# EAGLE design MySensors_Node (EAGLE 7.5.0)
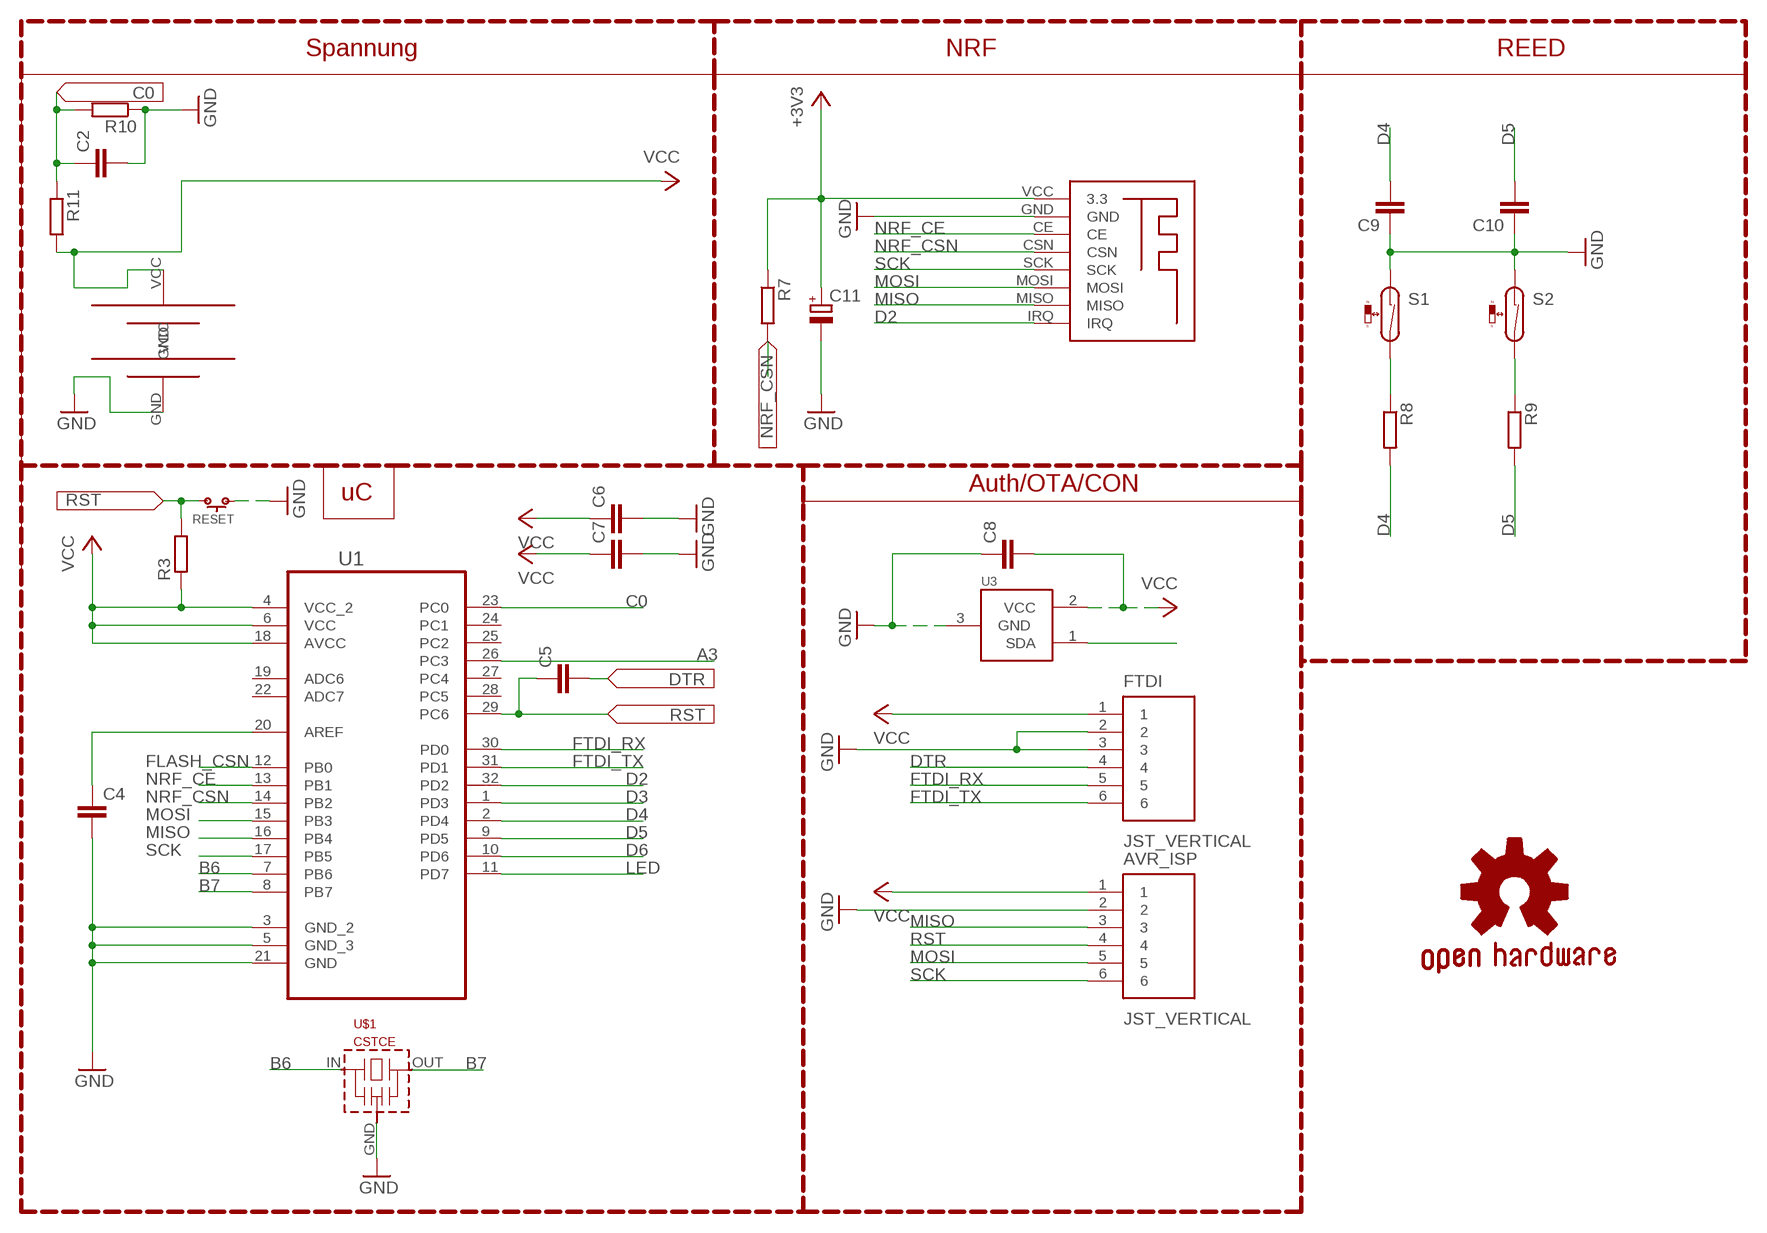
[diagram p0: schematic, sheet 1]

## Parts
AVR_ISP  JST_VERTICAL  [JST-6-SMD-VERT-1.0MM]
C2  C-EUC0805  [C0805]
C4  C-EUC0805  [C0805]
C5  C-EUC0805  [C0805]
C6  C-EUC0805  [C0805]
C7  C-EUC0805  [C0805]
C8  C-EUC0805  [C0805]
C9  C-EUC0805  [C0805]
C10  C-EUC0805  [C0805]
C11  CPOL-EUSANYO_SMD_C6  [SANYO-OSCON_SMD_C6]
FTDI  JST_VERTICAL  [JST-6-SMD-VERT-1.0MM]
GOLD_ORB_SM1  OSHWLOGO_GOLD_ORB_SM  [OSHW2]
R3  R-EU_R0805  [R0805]
R7  R-EU_R0805  [R0805]
R8  R-EU_R0805  [R0805]
R9  R-EU_R0805  [R0805]
R10  R-EU_R0805  [R0805]
R11  R-EU_R0805  [R0805]
RESET  SPST.B3U-1000P(M)  [B3U-1000P(M)]
S1  REED-SWITCH-MK6-5-C  [MK6-5]
S2  REED-SWITCH-MK6-5-C  [MK6-5]
U1  ATMEGA328P-AU  [QFP80P900X900X120-32N]
U3  IC_ATSHA204A_CRYPT  [SOT23-3]
U$1  CSTCE  [CSTCE]
U$2  NRF24SMD  [NRF24SMD]
U$3  AAA_HOLDER  [AAA_HOLDER]

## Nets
A3: U1.26(PC3) U3.1(SDA)
B6: U1.7(PB6) U$1.IN
B7: U1.8(PB7) U$1.OUT
C0: C2.1 R10.2 R11.1 U1.23(PC0)
D2: U1.32(PD2) U$2.IRQ
D3: U1.1(PD3)
D4: C9.2 R8.2 U1.2(PD4)
D5: C10.2 R9.2 U1.9(PD5)
D6: U1.10(PD6)
DTR: C5.2 FTDI.4
FLASH_CSN: U1.12(PB0)
FTDI_RX: FTDI.5 U1.30(PD0)
FTDI_TX: FTDI.6 U1.31(PD1)
GND: AVR_ISP.2 C2.2 C4.2 C6.2 C7.2 C8.1 C9.1 C10.1 C11.- FTDI.2 FTDI.3 R10.1 RESET.1 S1.1 S2.1 U1.3(GND_2) U1.5(GND_3) U1.21(GND) U3.3(GND) U$1.GND U$2.GND U$3.GND
LED: U1.11(PD7)
MISO: AVR_ISP.3 U1.16(PB4) U$2.MISO
MOSI: AVR_ISP.5 U1.15(PB3) U$2.MOSI
N$4: R8.1 S1.2
N$5: R9.1 S2.2
N$7: C4.1 U1.20(AREF)
NRF_CE: U1.13(PB1) U$2.CE
NRF_CSN: R7.2 U1.14(PB2) U$2.CSN
RST: AVR_ISP.4 C5.1 R3.2 RESET.2 U1.29(PC6)
SCK: AVR_ISP.6 U1.17(PB5) U$2.SCK
VCC: AVR_ISP.1 C6.1 C7.1 C8.2 C11.+ FTDI.1 R3.1 R7.1 R11.2 U1.4(VCC_2) U1.6(VCC) U1.18(AVCC) U3.2(VCC) U$2.VCC(3.3) U$3.VCC ; supply symbol labelled +3V3
Unconnected: U1.19(ADC6) U1.22(ADC7) U1.24(PC1) U1.25(PC2) U1.27(PC4) U1.28(PC5)

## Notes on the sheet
- Spannung | NRF | REED
- Auth/OTA/CON
- uC

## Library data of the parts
AVR_ISP FTDI = SparkFun-Connectors:JST_VERTICAL; PROD_ID: CONN-08249
C2 C4-C10 = rcl:C-EU: CAPACITOR, European symbol
C11 = rcl:CPOL-EU: POLARIZED CAPACITOR, European symbol
GOLD_ORB_SM1 = bfl:OSHWLOGO: These are Open-Source Hardware logos.
R3 R7-R11 = rcl:R-EU_: RESISTOR, European symbol
RESET = omron:SPST
S1 S2 = switch-reed:REED-SWITCH-: Reed Sensor; MF: MEDER; MPN: MK6-5-C; OC_FARNELL: 1079480
U1 = Atmel_By_element14_Batch_1-00:ATMEGA328P-AU: 8-bit Microcontroller with In-System Programmable Flash; MPN: ATMEGA328P-AU; OC_FARNELL: 1715486; OC_NEWARK: 14R4631; PACKAGE: TQFP-32; SUPPLIER: Atmel
U3 = TD-MySensors:IC_ATSHA204A_CRYPT
U$1 = murata-cstcc-cstce-cstcr-cstcv-resonators:CSTCE: Murata CSTCE Resonator - 3,2 x 1,3 mm
U$2 = NRF24_SMD:NRF24SMD
U$3 = Andi_lib:AAA_HOLDER

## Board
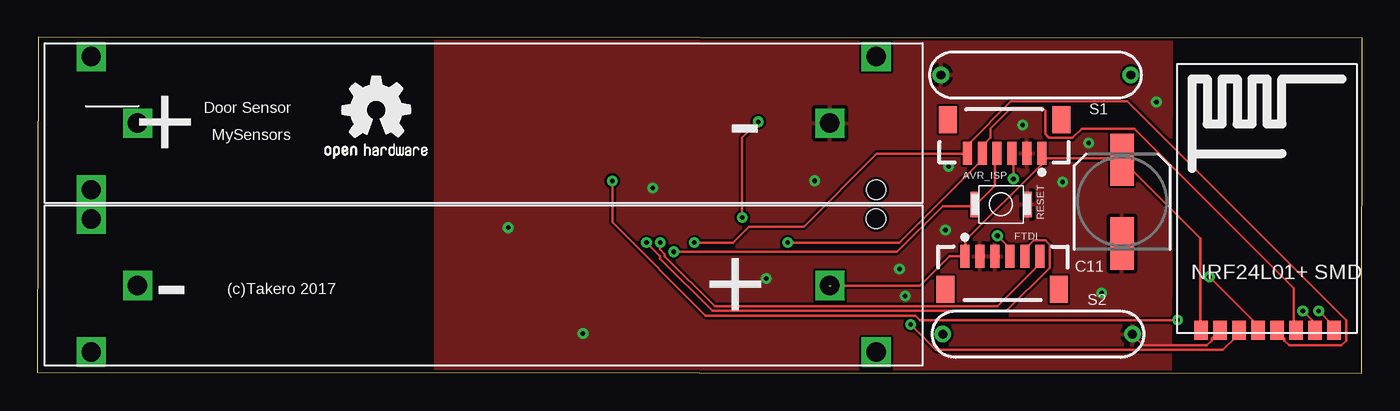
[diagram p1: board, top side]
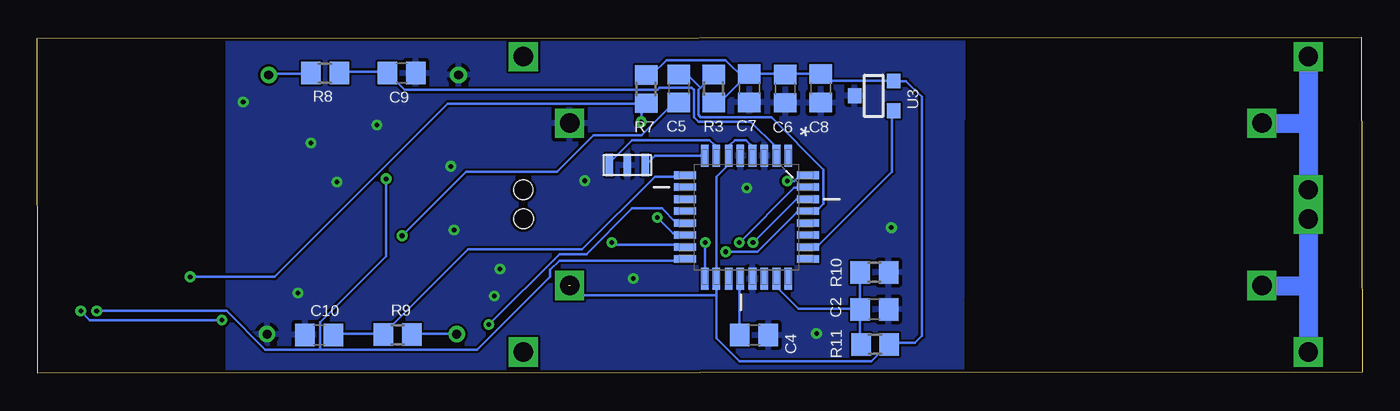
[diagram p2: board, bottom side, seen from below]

Size 88.6 x 22.47 mm. Coordinates in mm from the lower left corner, seen from the top.
Outline: 0.04,22.47 0,0.06 88.59,0 88.6,22.42 0.04,22.47
Copper layers (1*16): Top 0.035mm / dielectric 1.5mm / Bottom 0.035mm
Design rules "default *": minimum track width 6mil, minimum drill 12mil, track to track 6mil, track to pad 6mil, pad to pad 6mil, via to via 6mil, smd to smd 6mil, copper to edge 8mil, drill to drill 4mil, minimum pad ring 10mil, minimum via ring 8mil, stop-mask expansion 4mil, vias tented up to drill 12mil, thermal gap 10mil

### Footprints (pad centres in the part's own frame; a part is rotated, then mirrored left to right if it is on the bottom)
JST-6-SMD-VERT-1.0MM = smd 0.6 x 1.55: 1 -2.54,1.27; 2 -1.54,1.27; 3 -0.54,1.27; 4 0.46,1.27; 5 1.46,1.27; 6 2.46,1.27 | smd 1.2 x 1.8: P$1 -3.84,-0.955; P$2 3.76,-0.955
C0805 = smd 1.3 x 1.5: 1 -0.95,0; 2 0.95,0
SANYO-OSCON_SMD_C6 = smd 3.5 x 1.6: + 2.8,0; - -2.8,0
R0805 = smd 1.3 x 1.5: 1 -0.95,0; 2 0.95,0
B3U-1000P(M) = smd 0.6 x 1.7: 1 -1.75,0; 2 1.75,0
MK6-5 = drill 0.6 pad 1.016: 1 -6.35,0; 2 6.35,0
QFP80P900X900X120-32N = smd 1.473 x 0.508: 1 -4.115,2.794; 2 -4.115,2.007; 3 -4.115,1.194; 4 -4.115,0.406; 5 -4.115,-0.406; 6 -4.115,-1.194; 7 -4.115,-2.007; 8 -4.115,-2.794; 17 4.115,-2.794; 18 4.115,-2.007; 19 4.115,-1.194; 20 4.115,-0.406; 21 4.115,0.406; 22 4.115,1.194; 23 4.115,2.007; 24 4.115,2.794 | smd 0.508 x 1.473: 9 -2.794,-4.115; 10 -2.007,-4.115; 11 -1.194,-4.115; 12 -0.406,-4.115; 13 0.406,-4.115; 14 1.194,-4.115; 15 2.007,-4.115; 16 2.794,-4.115; 25 2.794,4.115; 26 2.007,4.115; 27 1.194,4.115; 28 0.406,4.115; 29 -0.406,4.115; 30 -1.194,4.115; 31 -2.007,4.115; 32 -2.794,4.115
SOT23-3 = smd 1 x 0.9: 1 -1,-1.3; 2 1,-1.3; 3 0,1.3
CSTCE = smd 0.5 x 1.5: GND 0,0; IN 1.2,0; OUT -1.2,0
NRF24SMD = smd 0.9 x 1.27: CE -1.27,-6.35; CSN 0,-6.35; GND -2.54,-6.35; IRQ 5.08,-6.35; MISO 3.81,-6.35; MOSI 2.54,-6.35; SCK 1.27,-6.35; VCC -3.81,-6.35
AAA_HOLDER = drill 1.3 pad 1.676 square: GND -5.35,27.75; P$1 5.5,-18.55; P$2 9.95,-21.65; P$3 1.05,-21.65; P$5 9.95,30.85; P$7 -5.35,-18.55; P$8 -0.9,-21.65; P$9 -9.8,-21.65; P$12 -9.8,30.85; VCC 5.5,27.75 | hole 1.3: -0.891,30.849; 1.051,30.842

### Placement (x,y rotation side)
AVR_ISP  64.65,16 180 top
C2  32.62,4.29 0 bottom
C4  40.66,2.56 0 bottom
C5  45.69,19.05 270 bottom
C6  38.58,19.05 270 bottom
C7  40.98,19.07 270 bottom
C8  36.2,19.05 90 bottom
C9  64.24,20.08 180 bottom
C10  69.75,2.57 0 bottom
C11  72.55,11.49 90 top
FTDI  64.57,6.57 0 top
GOLD_ORB_SM1  18.84,13.32 0 top
R3  43.37,19.05 90 bottom
R7  47.88,19.01 270 bottom
R8  69.37,20.08 0 bottom
R9  64.51,2.59 180 bottom
R10  32.62,6.75 180 bottom
R11  32.57,1.94 0 bottom
RESET  64.45,11.3 180 top
S1  66.78,19.95 0 top
S2  66.9,2.63 180 top
U1  41.18,10.45 270 bottom
U3  32.64,18.55 90 bottom
U$1  49.14,13.92 180 bottom
U$2  81.63,9.25 0 top
U$3  25.25,11.38 270 top

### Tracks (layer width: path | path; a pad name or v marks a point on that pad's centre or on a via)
A3
  Bottom 0.152: U3.1 31.44,17.43 31.44,13.47 36.32,8.59 36.93,8.59 U1.26
B6
  Bottom 0.152: U1.7 43.33,14.69 43.33,15.3 43.63,15.6 48.82,15.6 50.19,14.23 50.19,13.93 U$1.IN
B7
  Bottom 0.152: U1.8 44.09,14.54 47.29,14.54 47.9,13.93 U$1.OUT
C0
  Bottom 0.152: 33.58,4.33 37.69,4.33 39.06,5.7 39.06,6.31 U1.23 | R11.1 33.58,2.04 33.58,4.17 C2.1 33.58,4.33 | 33.58,4.33 33.58,6.61 R10.2
D2  (via drill 0.3)
  Top 0.152: v85.7,4.17 86.61,3.26 86.61,2.95 U$2.IRQ | v76.25,3.56 59.03,3.56 58.72,3.87 44.7,3.87 38.45,10.12 v38.45,12.86
  Bottom 0.152: v85.7,4.17 85.09,3.56 v76.25,3.56 | v38.45,12.86 37.99,12.86 37.69,13.16 37.08,13.16 U1.32
D4
  Bottom 0.152: U1.2 39.21,14.69 39.21,15.15 40.89,16.82 44.4,16.82 44.7,17.13 44.7,18.96 44.85,19.11 46.99,19.11 47.14,18.96 64.06,18.96 65.12,20.02 C9.2 65.27,20.18 68.32,20.18 R8.2
D5
  Bottom 0.152: U1.9 45.31,13.16 47.29,13.16 52.17,8.29 59.79,8.29 65.43,2.65 R9.2 65.58,2.65 68.78,2.65 C10.2
DTR  (via drill 0.3)
  Top 0.152: v64.21,9.2 64.97,8.44 64.97,7.98 FTDI.4
  Bottom 0.152: v64.21,9.2 59.94,13.47 53.84,13.47 51.41,15.91 48.21,15.91 46.07,18.04 45.77,18.04 C5.2
FTDI_RX  (via drill 0.3)
  Top 0.152: v40.74,8.75 41.65,7.83 41.65,7.68 45.16,4.17 64.82,4.17 67.71,7.07 67.71,8.59 67.41,8.9 66.65,8.9 66.04,8.29 66.04,7.98 FTDI.5
  Bottom 0.152: v40.74,8.75 37.84,11.64 37.08,11.64 U1.30
FTDI_TX  (via drill 0.3)
  Top 0.152: v41.65,8.75 41.65,8.29 41.96,7.98 41.96,7.83 45.31,4.48 64.21,4.48 66.95,7.22 66.95,7.83 FTDI.6
  Bottom 0.152: v41.65,8.75 37.99,12.4 37.08,12.4 U1.31
GND  (via drill 0.3)
  Top 0.152: U$2.GND 78.99,2.8 78.53,2.34 78.53,2.19 78.23,1.89 73.96,1.89 73.35,2.5 S2.1 | 63.14,7.83 FTDI.2
  Bottom 0.152: C7.2 41.04,18.19 41.1,18
  other vias: 36.49,2.68 31.48,9.74 41.15,12.4 51.98,12.88 68.57,12.8 74.83,18.15 70.3,15.39 65.89,16.61 71.19,5.39 60.94,13.85 60.73,9.6 57.66,6.97 48.75,6.35 58.04,5.18
  pour Bottom: 26.76,22.9 26.84,-0.95 75.79,-1.11 75.81,23.1
  pour Top: 26.64,22.92 26.64,-0.71 75.76,-0.96 75.83,23.16
MISO  (via drill 0.3)
  Top 0.152: v84.63,4.17 85.39,3.41 85.39,2.95 U$2.MISO | v65.27,13.01 65.27,14.69 AVR_ISP.3
  Bottom 0.152: v84.63,4.17 75.94,4.17 73.35,1.58 69.69,1.58 | 69.69,1.58 59.18,1.58 54.3,6.46 54.3,6.92 53.69,7.53 45.31,7.53 U1.16 | v65.27,13.01 65.27,7.83 69.69,3.41 69.69,1.58
MOSI  (via drill 0.3)
  Top 0.152: U$2.MOSI 84.02,2.95 84.02,5.7 73.35,16.37 69.85,16.37 69.24,15.76 69.23,15.76 67.66,15.76 67.4,16.02 67.4,17.55 67.2,17.75 65.14,17.75 63.75,16.36 63.75,15.76 63.29,15.3 63.29,14.84 AVR_ISP.5 63.14,14.69 63.14,14.23 57.65,8.75 v50.19,8.75
  Bottom 0.152: v50.19,8.75 50.03,8.59 45.31,8.59 U1.15
N$2
  Bottom 1.27: 3.59,21.18 3.6,21.18 3.6,1.43
N$3
  Bottom 1.27: 6.7,16.71 3.62,16.71 3.62,16.69
N$4
  Bottom 0.152: R8.1 70.46,20.02 73.05,20.02 S1.2
N$5
  Bottom 0.152: R9.1 63.45,2.65 60.55,2.65 S2.2
N$6
  Bottom 1.27: 6.7,5.87 3.66,5.87
N$7
  Bottom 0.152: U1.20 41.65,6.31 41.65,2.65 C4.1
NRF_CE  (via drill 0.3)
  Top 0.152: v58.42,3.26 60.09,1.58 79.3,1.58 80.21,2.5 80.21,2.8 U$2.CE
  Bottom 0.152: v58.42,3.26 53.69,7.98 51.86,7.98 48.82,11.03 46.83,11.03 45.92,10.12 45.31,10.12 U1.13
NRF_CSN  (via drill 0.3)
  Top 0.152: v78.38,6.46 81.58,3.26 81.58,2.95 U$2.CSN | v47.14,10.42 47.14,15.76 v48.21,16.82
  Bottom 0.152: v78.38,6.46 72.74,6.46 61.16,18.04 48.21,18.04 | 48.21,18.04 47.9,18.04 R7.2 48.21,18.04 | v47.14,10.42 46.07,9.35 45.31,9.35 U1.14 | 48.21,18.04 v48.21,16.82
RST  (via drill 0.3)
  Top 0.152: AVR_ISP.4 64.06,14.69 64.06,12.56 62.84,11.34 RESET.2 62.68,11.18 60.55,11.18 57.5,8.14 v42.57,8.14
  Bottom 0.152: 44.24,19.11 43.48,19.87 R3.2 | 44.24,19.11 44.4,18.96 44.4,17.28 44.24,17.13 39.52,17.13 36.01,13.62 36.01,11.34 36.47,10.88 36.93,10.88 U1.29 37.08,10.73 37.84,10.73 40.43,8.14 v42.57,8.14 | 44.24,19.11 45.01,19.87 45.61,19.87 C5.1
SCK  (via drill 0.3)
  Top 0.152: U$2.SCK 82.95,2.8 83.41,2.34 83.41,2.19 83.71,1.89 87.22,1.89 87.52,2.19 87.52,3.56 72.89,18.19 65.12,18.19 62.23,15.3 62.23,14.84 AVR_ISP.6 62.07,14.69 56.13,14.69 51.25,9.81 47.6,9.81 46.53,8.75 v43.94,8.75
  Bottom 0.152: v43.94,8.75 43.94,6.46 U1.17
VCC  (2 unrouted)
  Top 0.152: U$2.VCC 77.77,2.95 77.77,9.05 72.59,14.23 C11.+ 72.44,14.38 67.1,14.38 | 67.1,14.38 67.1,14.69 AVR_ISP.1 67.1,14.38 | 67.1,14.38 67.1,13.93 62.07,8.9 62.07,7.98 FTDI.1 61.92,7.83 61.01,7.83 59.03,5.85 53.08,5.85
  Bottom 0.152: U3.2 31.44,19.57 35.86,19.57 36.17,19.87 C8.2 36.32,20.02 38.45,20.02 C6.1 38.6,20.02 40.89,20.02 C7.1 | 41.35,19.72 41.04,20.02 C7.1 | 41.35,19.72 42.87,18.19 43.33,18.19 R3.1 | 41.35,19.72 42.57,20.94 46.53,20.94 47.44,20.02 47.75,20.02 R7.1 | 41.35,19.72 C7.1 | U1.4 40.89,14.69 40.89,15.3 41.2,15.6 41.96,15.6 42.26,15.3 42.26,14.69 U1.6 42.41,14.54 42.41,13.93 43.18,13.16 43.18,6.46 U1.18 43.18,6.31 43.18,5.24 | 43.18,5.24 43.18,2.34 41.65,0.82 32.81,0.82 31.75,1.89 R11.2 31.59,2.04 29.9,2.04 29.43,2.5 29.43,18.49 30.49,19.55 U3.2 | 31.29,19.41 U3.2 | 43.18,5.24 52.47,5.24 52.93,5.7 52.93,5.85

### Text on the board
tPlace: Door Sensor | MySensors | (c)Takero 2017
tNames: + | - | - | +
